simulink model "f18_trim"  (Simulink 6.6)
settings: Solver=ode45  StartTime=0.0  StopTime=10.0  RelTol=1e-3

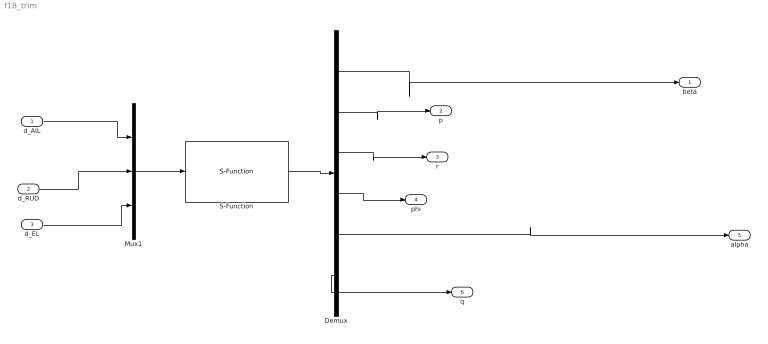
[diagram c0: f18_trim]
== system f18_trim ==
  d_AIL : Inport
  d_RUD : Inport  Port=2
  d_EL : Inport  Port=3
  Demux : Demux  Outputs=6
  Mux1 : Mux  Inputs=3
  S-Function : S-Function  FunctionName=f18_sfcn  Parameters=x_init
  beta : Outport
  p : Outport  Port=2
  r : Outport  Port=3
  phi : Outport  Port=4
  alpha : Outport  Port=5
  q : Outport  Port=6
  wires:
  Mux1/1 -> S-Function/1
  S-Function/1 -> Demux/1
  Demux/1 -> beta/1
  Demux/5 -> alpha/1
  Demux/2 -> p/1
  Demux/6 -> q/1
  Demux/3 -> r/1
  Demux/4 -> phi/1
  d_AIL/1 -> Mux1/1
  d_EL/1 -> Mux1/3
  d_RUD/1 -> Mux1/2
